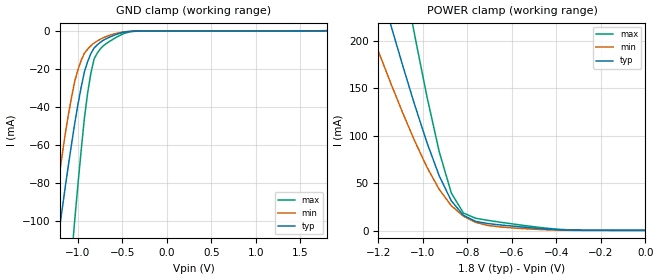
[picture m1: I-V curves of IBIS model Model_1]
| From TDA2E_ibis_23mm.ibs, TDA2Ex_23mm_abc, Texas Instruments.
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| Model based on original model for BMLBLVDS18_SSCEH
|   Sub model LVDS_RX_MODE_5P_1P8
[model]   Model_1
|[Description]  [1.8V-INPUT-LVDS MODE-X, IND, 5%]
|   LVDS MODE,IND,5%
|[Input Load]   LVDS MODE
|[Output Drive]
|Voltage   1.8V
|Mode   INPUT
Model_type   Input
Polarity   Non-Inverting
Vinl =  1.15V
Vinh =  1.25V
C_comp   3.4p   3.05p   3.82p
[Temperature Range]   25   125   -40
[Voltage Range]   1.8   1.71   1.89
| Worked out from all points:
|   GND clamp passes 1 mA (typ) near -0.51 V on its own axis
|   POWER clamp passes 1 mA (typ) near -0.40 V on its own axis
[POWER_clamp]
-1.8V     779.9mA    580mA      1.224A
-1.236V   292.1mA    211mA      460.4mA
-1.145V   217.2mA    155.6mA    341.7mA
-1.127V   202.7mA    145mA      318.5mA
-1.055V   145.7mA    103.9mA    227.2mA
-1.036V   131.7mA    93.92mA    204.8mA
-927.3mV  57.78mA    43.44mA    83.3mA
-872.7mV  31.31mA    26.16mA    39.59mA
-818.2mV  16.05mA    15.09mA    18.44mA
-709.1mV  7.358mA    5.377mA    10.73mA
-600mV    4.702mA    2.805mA    7.054mA
0V        145uA      60.2uA     263.6uA
[GND_clamp]
-1.8V     -321.4mA   -309.3mA   -563.6mA
-1.291V   -133.4mA   -105mA     -247.8mA
-1.218V   -107.9mA   -79mA      -204.2mA
-1.073V   -59.81mA   -35.07mA   -120mA
-1.036V   -48.68mA   -26.51mA   -99.87mA
-927.3mV  -21.51mA   -11.72mA   -45.84mA
-890.9mV  -16.08mA   -9.549mA   -32.59mA
-818.2mV  -8.944mA   -6.334mA   -14.72mA
-781.8mV  -7.267mA   -5.252mA   -11.57mA
-600mV    -2.366mA   -1.611mA   -4.175mA
-381.8mV  -124.6uA   -115.9uA   -225uA
1.8V      145uA      89.85uA    222.6uA
